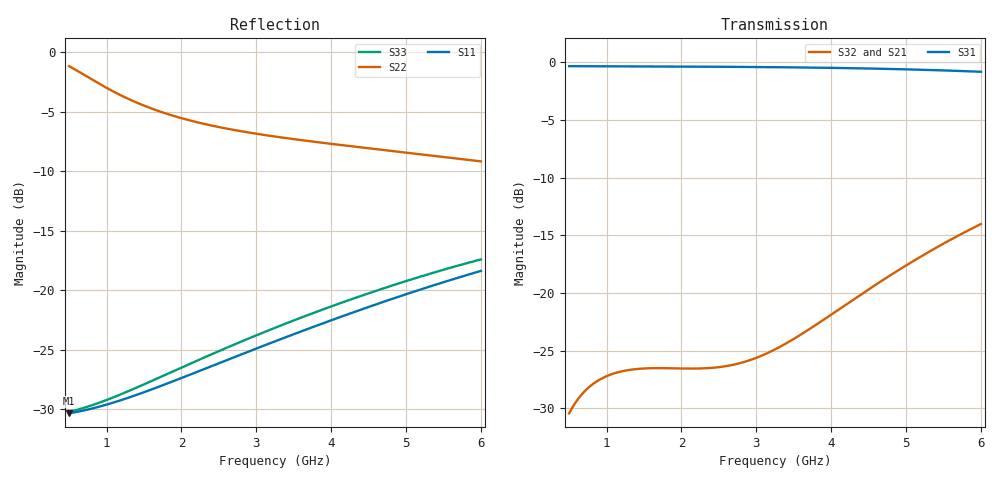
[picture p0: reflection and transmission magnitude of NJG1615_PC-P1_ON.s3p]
! NJG1615HA8(SPDT switch) S-parameter(S3P)/touchstone format
! P1-PC thru mode
! Port1...P1 terminal  Port2...P2 terminal  Port3...PC terminal
! VCTL(H)=3.0V  VCTL(L)=0V
! freq = 0.5GHz - 6GHz  10MHz step
# hz S ma R 50
! 3 Port Network Data from SP1.SP block
! freq  magS11  angS11  magS12  angS12  magS13  angS13
!  magS21  angS21
!  magS22  angS22  magS23  angS23
!  magS31  angS31  magS32  angS32
!  magS33  angS33
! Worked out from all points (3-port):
!   551 points, 500 MHz to 6 GHz, reference 50 ohm
!   strongest paths, dB at 500 MHz, 1.87 GHz, 3.25 GHz, 4.63 GHz, 6 GHz:
!     S31: -0.3, -0.4, -0.4, -0.5, -0.8
!     S32: -30.4, -26.5, -24.9, -19.1, -14.0
!     S21: -30.7, -26.8, -25.2, -19.5, -14.4
!   lowest |S11| = -30.4 dB at 500 MHz (marker M1), VSWR 1.06, Z = 52.9 - j1.11 ohm
!   |S11| at or under -10 dB: start of sweep to end of sweep
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5e8  0.03035 -20.2  0.02929 58.6  0.9635 -3.5
     0.02929 58.6  0.8751 -53.0  0.03003 59.0
     0.9635 -3.5  0.03003 59.0  0.03079 -21.7
7.3e8  0.03137 -28.6  0.03713 50.6  0.963 -5.0
       0.03713 50.6  0.7941 -73.2  0.03806 51.2
       0.963 -5.0  0.03806 51.2  0.03224 -30.4
1.01e9  0.03308 -38.1  0.04259 43.8  0.9623 -6.9
        0.04259 43.8  0.7065 -94.2  0.04365 44.6
        0.9623 -6.9  0.04365 44.6  0.03462 -40.0
1.26e9  0.03503 -46.0  0.04495 40.2  0.9617 -8.7
        0.04495 40.2  0.6442 -110.3  0.04607 41.1
        0.9617 -8.7  0.04607 41.1  0.03725 -47.7
1.54e9  0.03762 -54.2  0.04592 38.4  0.9611 -10.6
        0.04592 38.4  0.5905 -126.1  0.04706 39.6
        0.9611 -10.6  0.04706 39.6  0.04068 -55.3
2.27e9  0.04613 -72.8  0.04584 43.7  0.9588 -15.6
        0.04584 43.7  0.5032 -159.7  0.04703 45.5
        0.9588 -15.6  0.04703 45.5  0.05153 -71.9
3.25e9  0.06094 -93.6  0.05509 64.2  0.9538 -22.5
        0.05509 64.2  0.4426 164.3  0.05687 66.7
        0.9538 -22.5  0.05687 66.7  0.06948 -89.4
4.63e9  0.08781 -119.5  0.1064 77.2  0.9395 -32.5
        0.1064 77.2  0.3909 119.7  0.1104 80.4
        0.9395 -32.5  0.1104 80.4  0.1001 -110.9
5.31e9  0.1034 -131.7  0.1454 74.8  0.9275 -37.5
        0.1454 74.8  0.3692 97.7  0.151 78.2
        0.9275 -37.5  0.151 78.2  0.117 -121.2
6e9  0.1205 -144.2  0.1915 69.0  0.9111 -42.6
     0.1915 69.0  0.3482 74.7  0.199 72.8
     0.9111 -42.6  0.199 72.8  0.1347 -131.9
